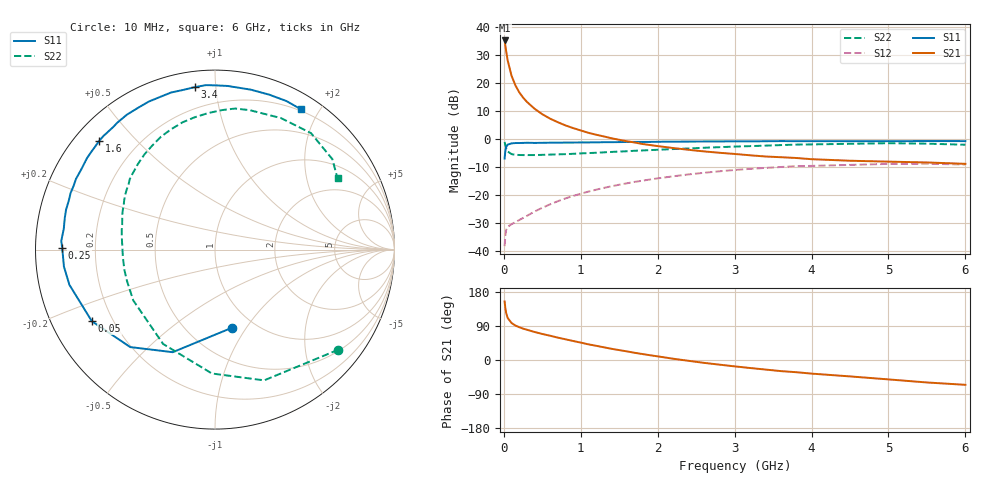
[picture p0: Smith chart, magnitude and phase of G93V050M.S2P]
! SIEMENS Small Signal Semiconductors
! BFG235
! Si NPN RF Bipolar Junction Transistor in SOT223
! VCE = 3 V  IC = 50 mA
! Common Emitter S-Parameters:  July  1994
# GHz  S  MA  R  50
!  f  S11  S21  S12  S22
! GHz  MAG  ANG  MAG  ANG  MAG  ANG  MAG  ANG
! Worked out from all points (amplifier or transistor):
!   40 points, 10 MHz to 6 GHz, reference 50 ohm
!   highest |S21| = 35.3 dB at 10 MHz (marker M1)
!   |S21| within 3 dB of that: start of sweep to 25.81 MHz
!   unconditionally stable (mu >= 1): 495 MHz to 1.413 GHz
!   at 200 MHz: K = 0.68, MSG = 22.9 dB, |S12| = -29.0 dB
!   at 1.5 GHz: K = 0.99, MSG = 8.1 dB, |S12| = -16.4 dB
!   at 6 GHz: K = 0.93, MSG = 0.1 dB, |S12| = -9.1 dB
!   S11 on the Smith chart (normalised r, x): 10 MHz: 0.79, -0.86; 50 MHz: 0.12, -0.27; 250 MHz: 0.08, +0.01; 1.6 GHz: 0.07, +0.39; 3.4 GHz: 0.08, +0.88; 6 GHz: 0.18, +1.78
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0.01  0.446 -78.1  58.43 154.6  0.012 67.1  0.8848 -39.1
0.02  0.6182 -112.4  47.03 136.3  0.019 50.2  0.7782 -69.4
0.03  0.7197 -131.0  37.71 124.2  0.0234 40.7  0.6906 -91.4
0.05  0.7937 -149.8  25.56 110.9  0.0266 31.7  0.6 -118.8
0.1  0.8346 -166.4  13.63 97.6  0.0298 29.2  0.5363 -148.1
0.15  0.847 -173.6  9.177 91.0  0.0323 33.0  0.5206 -160.3
0.2  0.8477 -177.5  6.876 86.6  0.0353 36.8  0.5174 -167.2
0.25  0.8516 179.3  5.54 82.8  0.0384 40.3  0.5149 -171.8
0.3  0.8578 176.8  4.63 79.9  0.0419 43.6  0.5151 -175.6
0.4  0.8505 172.1  3.483 73.9  0.0502 47.8  0.5158 179.2
0.5  0.8552 168.2  2.782 68.7  0.0585 50.4  0.5199 175.1
0.6  0.8591 165.0  2.323 64.1  0.0674 51.6  0.5254 171.4
0.7  0.8591 161.5  2.005 59.1  0.0766 52.2  0.5309 168.1
0.9  0.864 155.9  1.571 50.2  0.0953 51.3  0.5429 162.2
1.1  0.8687 149.3  1.29 41.3  0.1142 49.3  0.5597 156.5
1.6  0.885 136.8  0.913 22.7  0.1607 40.9  0.6034 142.9
2.2  0.8979 123.1  0.689 3.4  0.2144 28.6  0.6602 126.6
3.2  0.9071 101.3  0.511 -21.1  0.2915 5.2  0.7454 98.9
3.4  0.9121 97.1  0.486 -25.2  0.3032 0.3  0.7609 93.1
4.5  0.9132 77.4  0.408 -43.3  0.3435 -25.2  0.8199 63.3
5.5  0.9184 64.3  0.38 -59.3  0.3602 -47.2  0.8255 37.6
6  0.9168 58.4  0.359 -65.5  0.3492 -55.5  0.7899 30.2
